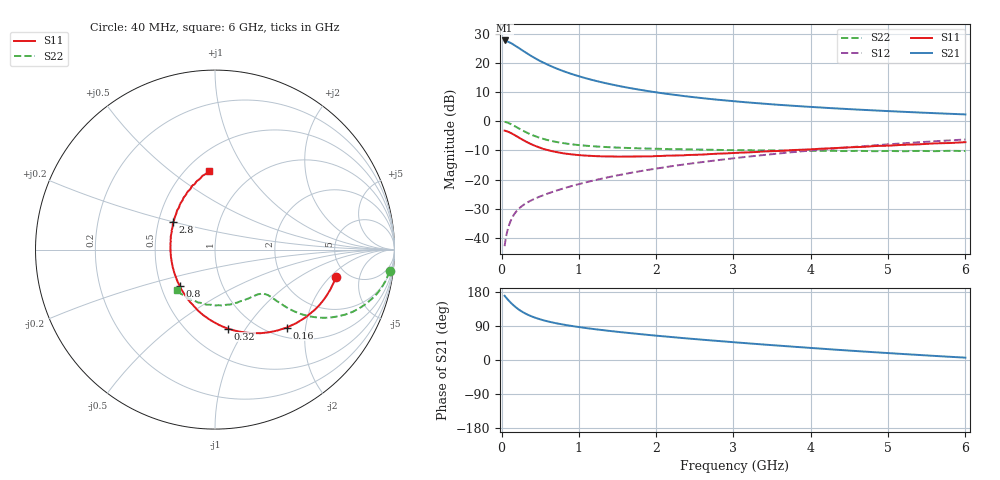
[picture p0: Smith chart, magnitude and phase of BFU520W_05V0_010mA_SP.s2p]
! Filename:  P:\Prog\Test\Noise\ATS_data\Testdata_Net\Run2\BFU520W_APM2013_06_A05_05p0V_010mA_SP_CM01_D.s2p
! Date/Time: Tue 26/Mar/2013 18:01:41
! BFU520W_APM2013_06_A05_05p0V_1to20mA_SP_CM01_Bias6_R.s2p
! MDIF S-parameter v. bias file
! BFU520W_APM2013_06_A05_05p0V_1to20mA_SP_CM01
! Date/time Thu Mar 21 14:22:37 2013
! VAR V_out= 5.0000
! VAR I_out= 10.0000
! VAR V_in= 0.8400
! VAR I_in= 0.1136
! Device data file deembeded for feedlines and parallel
! Original file: \Run2\BFU520W_APM2013_06_A05_05p0V_010mA_SP_CM01_R.s2p
! Feed-files: PR019V01_070313_Feed1.s2p, PR019V01_070313_Feed2.s2p
! Parallel-file: PR019V01_070313_Par.s2p
# MHz S MA R 50
!  Freq-MHz  S11-mag  S11-arg  S21-mag  S21-arg  S12-mag  S12-arg  S22-mag  S22-arg
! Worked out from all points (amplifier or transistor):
!   98 points, 40 MHz to 6 GHz, reference 50 ohm
!   highest |S21| = 27.8 dB at 40 MHz (marker M1)
!   |S21| within 3 dB of that: start of sweep to 247.1 MHz
!   unconditionally stable (mu >= 1): 1.427 GHz to 2.629 GHz
!   at 300 MHz: K = 0.52, MSG = 26.1 dB, |S12| = -28.4 dB
!   at 1.6 GHz: K = 1.01, MAG = 14.3 dB, |S12| = -18.1 dB
!   at 6 GHz: K = 0.87, MSG = 4.3 dB, |S12| = -6.3 dB
!   S11 on the Smith chart (normalised r, x): 40 MHz: 4.02, -2.35; 160 MHz: 1.19, -1.58; 320 MHz: 0.76, -0.83; 800 MHz: 0.62, -0.27; 2.8 GHz: 0.60, +0.20; 6 GHz: 0.64, +0.69
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40  0.6905 -12.8  24.45 169.5  0.007175 83.3  0.9798 -7.1
50  0.6856 -15.9  24.38 167.0  0.008866 82.3  0.973 -8.8
80  0.666 -25.3  23.41 159.9  0.01382 78.5  0.9458 -13.8
100  0.6491 -31.1  22.72 155.4  0.01687 76.1  0.9213 -16.8
120  0.6298 -36.9  22.11 151.1  0.01973 73.8  0.8962 -19.6
160  0.59 -47.4  20.53 143.5  0.02489 70.1  0.8413 -24.4
220  0.5301 -61.5  18.3 133.7  0.03115 66.5  0.7591 -29.7
280  0.4765 -73.5  16.18 125.8  0.03632 64.2  0.6873 -33.4
320  0.4458 -80.7  14.96 121.4  0.03938 63.3  0.6462 -35.2
400  0.3963 -93.0  12.87 114.2  0.04489 62.5  0.5793 -37.4
500  0.3516 -105.9  10.84 107.3  0.05131 62.6  0.5185 -38.8
550  0.3325 -111.6  10.06 104.3  0.05435 62.9  0.4942 -39.2
650  0.3078 -121.5  8.731 99.5  0.06074 63.6  0.4588 -39.6
800  0.2819 -134.3  7.271 93.5  0.07032 64.7  0.422 -40.1
1050  0.2599 -151.3  5.681 85.5  0.08677 66.2  0.3851 -40.9
1500  0.2477 -173.8  4.088 74.4  0.1179 67.0  0.3539 -44.3
2050  0.2534 166.6  3.074 63.3  0.1578 66.2  0.3367 -50.5
2800  0.2781 146.6  2.344 50.2  0.2153 63.1  0.3228 -62.2
3100  0.2898 139.9  2.156 45.4  0.2397 61.4  0.3203 -67.2
4100  0.3367 121.6  1.735 30.4  0.3239 54.6  0.3104 -87.2
5200  0.3951 104.9  1.456 15.7  0.4195 45.2  0.3065 -112.4
6000  0.4383 94.3  1.312 6.2  0.4868 37.5  0.3089 -132.8
